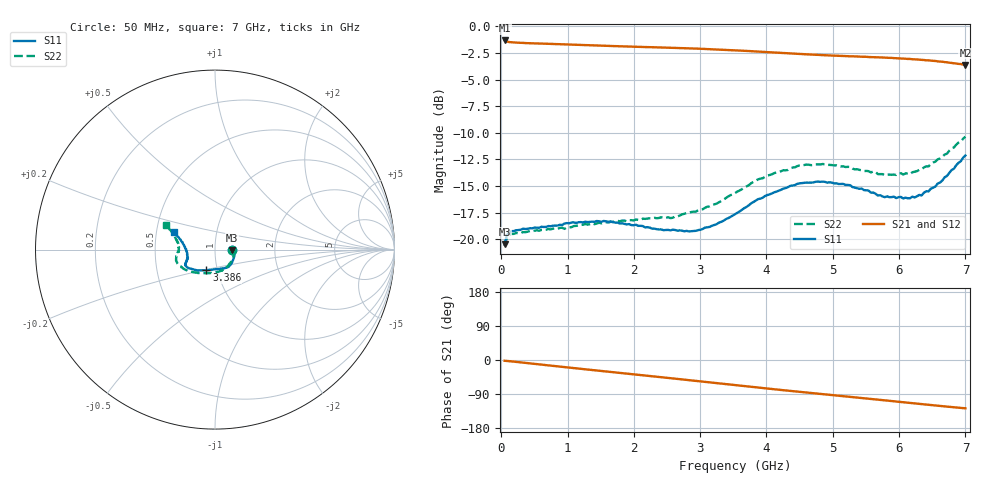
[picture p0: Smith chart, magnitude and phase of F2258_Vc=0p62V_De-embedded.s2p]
! Integrated Device Technology
! Corporate Headquarters
! 6024 Silver Creek Valley Road
! San Jose, CA 95138  USA
! Phone:  1-408-284-8200
! Toll Free:  1-800-223-1366
! Webpage:  http://www.idt.com/
! Timing and RF Division
! 515 Groton Road, Suite 102
! Westford, MA 01886-6024
! Device:  F2258
! Description: Voltage Variable RF Attenuator
! Frequency:  50.0 -  6000.00 MHz
! Package:  3x3 mm Thin QFN Plastic Package: 16 pin
! Ports:  2 RF, 2 DC
!  Pin  1  = NC
!  Pin  2  = NC
!  Pin  3  = RF2  = Port 2
!  Pin  4  = GND
!  Pin  5  = Vdd
!  Pin  6  = NC
!  Pin  7  = VCTRL
!  Pin  8  = NC
!  Pin  9  = GND
!  Pin 10  = RF1  = Port 1
!  Pin 11  = NC
!  Pin 12  = NC
!  Pin 13  = NC
!  Pin 14  = NC
!  Pin 15  = NC
!  Pin 16  = NC
! Vcntrl:  0.620 Volts
! Vdd:  +3.300 Volts
! Current:  1.111 mA
! Data:  The device was measured on a the F2258 evaluation board which has
!  individual transmission lines to the RF pins.  Data was collected
!  using a calibrated network analyzer.  The evaluation board was
!  de-embedded using a TRL calibration technique.
!  The reference plane is the edge of the package pin.
! Misc:  SN 10
!  Action Tracker AT0285
! Date Measured:  2014-12-10
! Date:  2016-01-13  MJV
! Note:
!  Integrated Device Technology supplies this data as a sample of measured
!  data at the package pin for this product.  Your particular data for this
!  product may vary.
!  Data was taken at 25 degrees C.
!  Integrated Device Technology reserves the right to change this data at anytime.
!Freq_(GHz)  S11M_(dB)  S11P_(deg)  S21M_(dB)  S21P_(deg)  S12M_(dB)  S12P_(deg)  S22M_(dB)  S22P_(deg)
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# GHz S dB R 50
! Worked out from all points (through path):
!   201 points, 50 MHz to 7 GHz, reference 50 ohm
!   highest |S21| = -1.33 dB at 50 MHz (marker M1); lowest = -3.6 dB at 7 GHz (marker M2)
!   group delay of S21, straight-line fit = 50.5 ps
!   lowest |S11| = -20.5 dB at 50 MHz (marker M3), VSWR 1.21, Z = 60.5 - j0.494 ohm
!   |S11| at or under -10 dB: start of sweep to end of sweep
!   |S22| runs from -20.6 to -10.4 dB; largest |S21 - S12| = 0.00059
!   S11 on the Smith chart (normalised r, x): 50 MHz: 1.21, -0.01; 3.386 GHz: 0.89, -0.21; 7 GHz: 0.62, +0.13
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0.05  -20.46 -2.4  -1.33 -2.0  -1.33 -2.0  -20.64 -2.7
0.08475  -19.60 -4.0  -1.44 -2.5  -1.44 -2.5  -19.81 -4.4
0.15425  -19.22 -6.3  -1.50 -3.7  -1.50 -3.7  -19.49 -7.6
0.71025  -18.75 -26.8  -1.65 -14.2  -1.64 -14.2  -19.03 -31.9
0.9535  -18.51 -36.3  -1.69 -18.8  -1.69 -18.8  -19.01 -43.7
1.2315  -18.41 -44.4  -1.76 -23.9  -1.76 -23.9  -18.63 -54.0
1.6485  -18.31 -54.3  -1.85 -31.5  -1.85 -31.5  -18.35 -67.0
2.37825  -19.07 -71.2  -1.98 -44.8  -1.98 -44.8  -17.99 -86.3
2.552  -19.15 -76.2  -2.02 -48.0  -2.01 -48.0  -18.00 -91.6
2.93425  -19.20 -91.3  -2.09 -55.1  -2.09 -55.1  -17.39 -105.3
3.386  -18.10 -112.5  -2.21 -63.6  -2.20 -63.6  -16.12 -123.7
3.525  -17.64 -118.4  -2.25 -66.3  -2.25 -66.3  -15.66 -128.9
4.0115  -15.84 -136.1  -2.43 -75.3  -2.43 -75.3  -14.01 -145.5
4.46325  -14.79 -146.4  -2.59 -83.5  -2.59 -83.5  -13.13 -157.3
4.7065  -14.65 -149.9  -2.66 -87.7  -2.66 -87.7  -13.02 -161.9
5.2625  -14.91 -156.1  -2.82 -97.4  -2.82 -97.4  -13.20 -170.6
5.6795  -15.89 -161.4  -2.91 -104.6  -2.91 -104.6  -13.87 -176.5
5.85325  -16.04 -165.4  -2.96 -107.7  -2.96 -107.7  -13.92 178.8
6.166  -16.14 -173.6  -3.07 -113.3  -3.07 -113.2  -13.86 172.3
6.33975  -15.87 179.0  -3.15 -116.4  -3.14 -116.4  -13.42 167.7
6.61775  -14.67 167.3  -3.31 -121.2  -3.31 -121.2  -12.40 160.9
7  -12.13 156.2  -3.62 -127.4  -3.63 -127.4  -10.36 153.0
